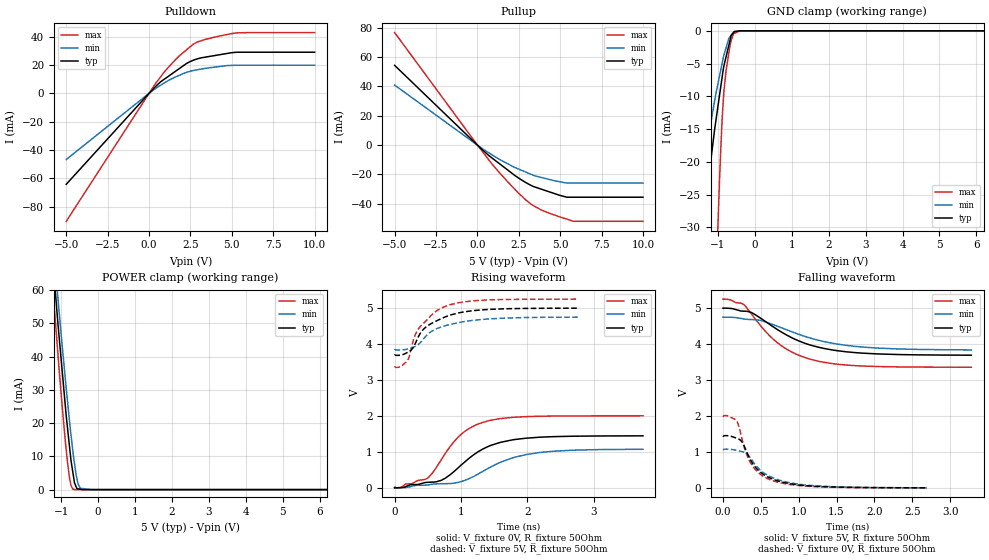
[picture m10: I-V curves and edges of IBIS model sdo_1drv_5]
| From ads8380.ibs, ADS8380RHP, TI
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|   sdo_1drv_5 Model
[Model]   sdo_1drv_5
Model_type   3-state
Polarity   Non-Inverting
Vmeas = 2.5
Vref = 2.5
Cref = 10pF
Rref = 50
|   typ   min   max
|   (nom PVT)   (fast PVT)   (slow PVT)
|C_comp from frequency sweep method (F=40MHz)
C_comp   5.189e-12   5.145e-12   5.197e-12
|ON state : BUFFER OUTPUT TURNED HIGH
|C_comp   4.901e-12   4.863e-12   4.902e-12
|OFF state: BUFFER IN HIGH IMPEDANCE
|C_comp   5.189e-12   5.145e-12   5.197e-12
|C_comp from LC tank measurement(L=1nH)
|Resonant Frequency(Hz)   4.120e+09   4.130e+09   4.110e+09
|C_comp   1.494e-12   1.487e-12   1.501e-12
|ON state : BUFFER OUTPUT TURNED HIGH
|Resonant Frequency(Hz)   4.120e+09   4.130e+09   4.110e+09
|C_comp   1.494e-12   1.487e-12   1.501e-12
|OFF state: BUFFER IN HIGH IMPEDANCE
|Resonant Frequency(Hz)   4.090e+09   4.100e+09   4.070e+09
|C_comp   1.516e-12   1.508e-12   1.531e-12
| Where nom  PVT is Nominal Process, 5V, 35C
|   Fast PVT is Strong Process,  5.25V, -40C
|   Slow PVT is Weak Process,   4.75V, 95C
[Voltage Range]   5   4.75   5.25
|Ambient Temperature   25   85   -40
|Junction Temperature
[Temperature Range]   35   95   -40
[Pullup Reference]   5   4.75   5.25
[Pulldown Reference]   0   0   0
[Power Clamp Reference]   5   4.75   5.25
[GND Clamp Reference]   0   0   0
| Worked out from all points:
|   slope of the pulldown table from 0 to 0.75 V, typ, clamps not added: 87.6 ohm
|   slope of the pullup table from 0 to 0.75 V, typ, clamps not added: 98.1 ohm
|   GND clamp passes 1 mA (typ) near -0.65 V on its own axis
|   POWER clamp passes 1 mA (typ) near -0.60 V on its own axis
|   falling waveform, V_fixture 5V, R_fixture 50Ohm: 20-80 % time 704ps typ, 824ps min, 588ps max; typ from 5 V to 3.69 V
|   rising waveform, V_fixture 0V, R_fixture 50Ohm: 20-80 % time 637ps typ, 758ps min, 520ps max; typ from 0 V to 1.44 V
|   rising waveform, V_fixture 5V, R_fixture 50Ohm: 20-80 % time 445ps typ, 512ps min, 363ps max; typ from 3.69 V to 5 V
|   falling waveform, V_fixture 0V, R_fixture 50Ohm: 20-80 % time 323ps typ, 392ps min, 257ps max; typ from 1.45 V to 0.007 V
[Pulldown]
|   Voltage   I(typ)   I(min)   I(max)
-5V       -64.14mA   -46.65mA   -90.25mA
420mV     5.095mA    3.675mA    7.376mA
924mV     10.01mA    7.353mA    15.1mA
1.596V    15.56mA    11.55mA    23.74mA
2.27V     21.14mA    14.82mA    30.79mA
2.672V    23.39mA    16.13mA    34.73mA
2.94V     24.44mA    16.69mA    36.35mA
3.433V    25.63mA    17.7mA     38.18mA
5.282V    28.97mA    19.9mA     42.66mA
10V       29.05mA    19.91mA    42.9mA
[GND Clamp]
|   Voltage   I(typ)   I(min)   I(max)
-5V       -615.5mA   -386.5mA   -1.626A
-1.64V    -41.74mA   -31.12mA   -149mA
-1.554V   -37.39mA   -27.67mA   -129.6mA
-1.31V    -25.06mA   -17.89mA   -83.47mA
-1.04V    -13.06mA   -9.152mA   -35.78mA
-955.5mV  -9.768mA   -6.844mA   -22.57mA
-892.5mV  -7.298mA   -5.113mA   -14.17mA
-840mV    -5.374mA   -3.735mA   -9.308mA
-777mV    -3.894mA   -2.533mA   -5.953mA
-677.3mV  -1.552mA   -932.8uA   -2.381mA
-565.3mV  -175.4uA   -114uA     -404uA
10V       0A         0A         0A
[Pullup]
|   Voltage   I(typ)   I(min)   I(max)
-5V       54.27mA    40.83mA    76.57mA
115.6fV   -27.52pA   -31.43pA   -20.94pA
924mV     -9.146mA   -6.921mA   -13.45mA
1.596V    -14.94mA   -11.35mA   -22.04mA
2.478V    -22.34mA   -16.26mA   -32.64mA
3.26V     -27.52mA   -19.96mA   -40.3mA
3.838V    -29.91mA   -21.99mA   -44.02mA
4.96V     -34.15mA   -24.93mA   -48.81mA
5.405V    -35.47mA   -25.85mA   -50.41mA
5.806V    -35.47mA   -25.85mA   -51.85mA
10V       -35.47mA   -25.85mA   -51.86mA
[POWER Clamp]
|   Voltage   I(typ)   I(min)   I(max)
-5V       1.111A     889.6mA    1.639A
-1.306V   79.05mA    85.45mA    71.92mA
-1.088V   49.82mA    57.38mA    40.53mA
-971.2mV  35.38mA    43.02mA    24.75mA
-829.5mV  18.56mA    26.58mA    8.235mA
-771.8mV  12.57mA    20.28mA    3.302mA
-687.7mV  5.414mA    11.93mA    186.9uA
-640mV    2.027mA    7.843mA    19.67uA
-546.3mV  251.2uA    1.859mA    2.402uA
-484.5mV  133.4uA    394.9uA    2.131uA
-190mV    0A         44.23nA    835.9nA
10V       0A         0A         0A
[Ramp]
R_load = 50
|   typ   min   max
dV/dt_r   0.871031/6.42996e-10   0.64614/7.63939e-10   1.20472/5.21094e-10
dV/dt_f   0.788082/7.12733e-10   0.549774/8.37436e-10   1.13806/5.92291e-10
[Falling Waveform]
V_fixture = 5V
V_fixture_min = 4.75V
V_fixture_max = 5.25V
R_fixture = 50Ohm
|   Time   V(typ)   V(min)   V(max)
0s        5V         4.75V      5.25V
272ps     4.917V     4.703V     5.107V
378ps     4.878V     4.685V     4.835V
566ps     4.623V     4.613V     4.344V
716ps     4.41V      4.502V     4.045V
926ps     4.162V     4.331V     3.764V
1.184ns   3.958V     4.152V     3.565V
1.46ns    3.834V     4.021V     3.456V
1.84ns    3.751V     3.921V     3.393V
3.28ns    3.694V     3.841V     3.359V
[Rising Waveform]
V_fixture = 0V
V_fixture_min = 0V
V_fixture_max = 0V
R_fixture = 50Ohm
|   Time   V(typ)   V(min)   V(max)
0s        7.028nV    11.9nV     6.362nV
96ps      4.202mV    1.122mV    12.06mV
504ps     152.8mV    78.83mV    279.2mV
710ps     212.2mV    112.5mV    797.9mV
952ps     544.1mV    147.4mV    1.396V
1.114ns   805.2mV    246.3mV    1.637V
1.334ns   1.081V     460.6mV    1.819V
1.78ns    1.332V     831.8mV    1.958V
2.174ns   1.404V     977mV      1.989V
3.746ns   1.444V     1.07V      2.001V
[Rising Waveform]
V_fixture = 5V
V_fixture_min = 4.75V
V_fixture_max = 5.25V
R_fixture = 50Ohm
|   Time   V(typ)   V(min)   V(max)
0s        3.686V     3.834V     3.353V
92ps      3.69V      3.832V     3.374V
196ps     3.768V     3.859V     3.539V
224ps     3.798V     3.874V     3.673V
294ps     3.944V     3.919V     4.171V
376ps     4.261V     4.013V     4.459V
550ps     4.563V     4.342V     4.792V
774ps     4.76V      4.511V     5.05V
1.394ns   4.957V     4.691V     5.223V
2.77ns    4.995V     4.745V     5.246V
[Falling Waveform]
V_fixture = 0V
V_fixture_min = 0V
V_fixture_max = 0V
R_fixture = 50Ohm
|   Time   V(typ)   V(min)   V(max)
0s        1.452V     1.078V     2.008V
182ps     1.383V     1.05V      1.864V
256ps     1.266V     1.012V     1.322V
306ps     1.042V     963.7mV    969mV
362ps     786.3mV    840.6mV    705.8mV
476ps     474.3mV    531mV      414.2mV
608ps     291.6mV    334mV      244.8mV
866ps     127.5mV    153.9mV    102.1mV
1.228ns   49.14mV    61.52mV    38.52mV
2.692ns   6.653mV    5.968mV    6.275mV
